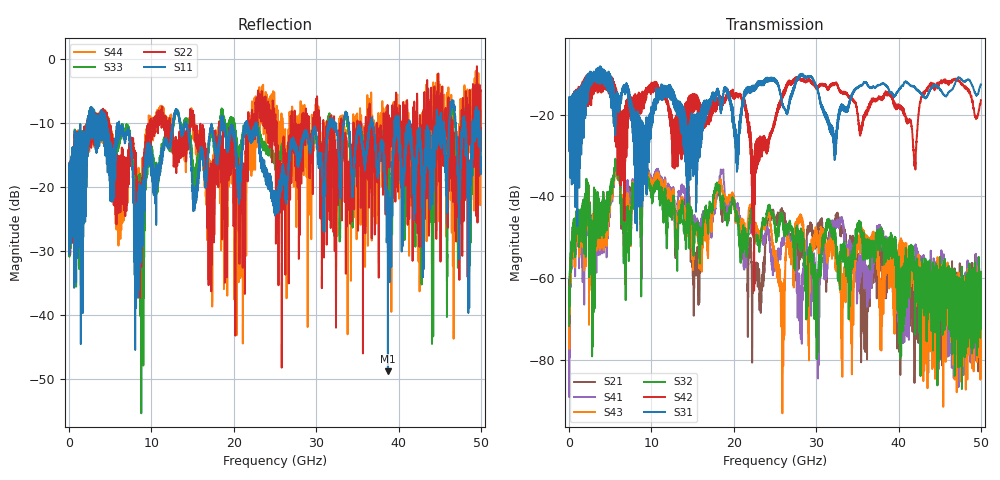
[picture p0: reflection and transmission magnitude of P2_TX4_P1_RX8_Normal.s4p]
!Keysight Technologies,N5225B,MY57041031,A.13.20.10
!Date: Friday, May 31, 2019 11:26:49
!Correction: S11(Full 4 Port(1,2,3,4))
!S12(Full 4 Port(1,2,3,4))
!S13(Full 4 Port(1,2,3,4))
!S14(Full 4 Port(1,2,3,4))
!S21(Full 4 Port(1,2,3,4))
!S22(Full 4 Port(1,2,3,4))
!S23(Full 4 Port(1,2,3,4))
!S24(Full 4 Port(1,2,3,4))
!S31(Full 4 Port(1,2,3,4))
!S32(Full 4 Port(1,2,3,4))
!S33(Full 4 Port(1,2,3,4))
!S34(Full 4 Port(1,2,3,4))
!S41(Full 4 Port(1,2,3,4))
!S42(Full 4 Port(1,2,3,4))
!S43(Full 4 Port(1,2,3,4))
!S44(Full 4 Port(1,2,3,4))
!S4P File: Measurements: <S11,S12,S13,S14>,
!<S21,S22,S23,S24>,
!<S31,S32,S33,S34>,
!<S41,S42,S43,S44>:
# Hz S  dB  R 50.0
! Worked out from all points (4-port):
!   5000 points, 10 MHz to 50 GHz, reference 50 ohm
!   strongest paths, dB at 10 MHz, 12.51 GHz, 25.01 GHz, 37.51 GHz, 50 GHz:
!     S31: -19.3, -14.3, -11.3, -12.8, -12.5
!     S42: -19.4, -24.3, -21.7, -16.2, -16.4
!     S32: -71.7, -43.2, -48.2, -53.1, -58.5
!     S43: -65.3, -40.2, -54.7, -54.6, -78.4
!     S41: -68.8, -39.3, -57.1, -48.6, -74.8
!     S21: -65.9, -42.6, -45.6, -58.6, -65.1
!   lowest |S11| = -48.8 dB at 38.71 GHz (marker M1), VSWR 1.01, Z = 49.6 + j0.0487 ohm
!   |S11| at or under -10 dB: 6.073 GHz to 12.61 GHz (6.542 GHz wide, 70 % of centre); 14.21 GHz to 18.43 GHz (4.227 GHz wide, 25.9 % of centre); 22.71 GHz to 31.52 GHz (8.804 GHz wide, 32.5 % of centre)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
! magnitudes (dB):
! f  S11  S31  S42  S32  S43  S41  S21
! 10 MHz  -19.0  -19.3  -19.4  -71.7  -65.3  -68.8  -65.9
! 5.74 GHz  -11.9  -17.2  -15.7  -32.7  -33.1  -33.2  -32.9
! 24.16 GHz  -18.6  -11.8  -27.1  -42.9  -44.3  -48.7  -45.8
! 25.91 GHz  -17.8  -17.3  -16.0  -45.1  -82.5  -50.5  -43.9
! 27.98 GHz  -14.7  -10.6  -11.2  -49.6  -45.5  -65.1  -52.2
! 38.71 GHz  -48.8  -13.5  -15.2  -53.1  -55.9  -51.0  -54.2
! 50 GHz  -15.3  -12.5  -16.4  -58.5  -78.4  -74.8  -65.1
